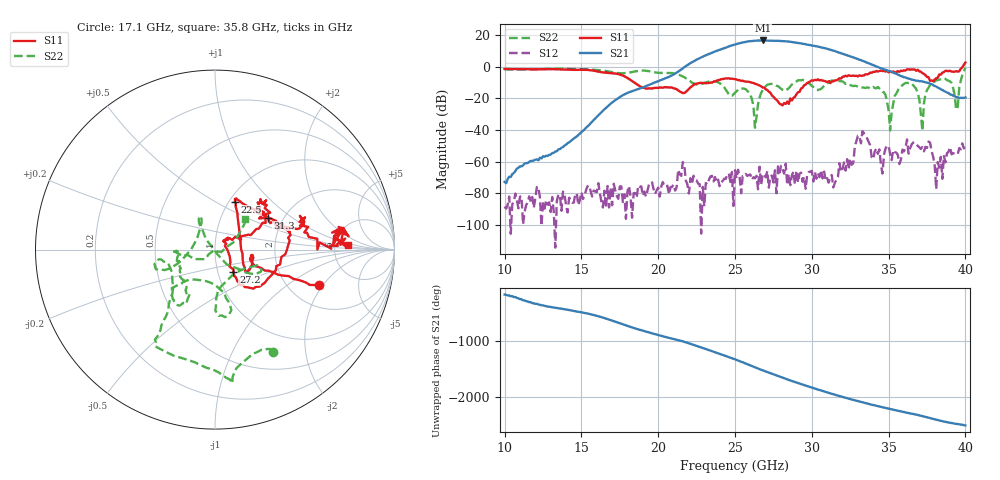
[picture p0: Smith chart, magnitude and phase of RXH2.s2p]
!Keysight Technologies,M9808A,MY58100618,A.14.70.03
!Date: Monday, February 27, 2023 13:24:29
!Correction: S11(Cdelta 2-Port  )
!S21(Cdelta 2-Port  )
!S12(Cdelta 2-Port  )
!S22(Cdelta 2-Port  )
!S2P File: Measurements: S11, S21, S12, S22:
# Hz S  RI  R 50
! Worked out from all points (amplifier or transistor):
!   301 points, 10 GHz to 40 GHz, reference 50 ohm
!   highest |S21| = 16.5 dB at 26.8 GHz (marker M1)
!   |S21| within 3 dB of that: 24.85 GHz to 29.92 GHz (5.075 GHz wide, 18.5 % of centre)
!   unconditionally stable (mu >= 1): start of sweep to 39.83 GHz
!   at 15 GHz: K = 61616.39, MAG = -31.9 dB, |S12| = -79.4 dB
!   at 25 GHz: K = 153.75, MAG = 14.8 dB, |S12| = -65.5 dB
!   at 40 GHz: K = -150.11, MSG = 15.3 dB, |S12| = -50.1 dB
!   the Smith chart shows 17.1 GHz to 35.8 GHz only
!   S11 on the Smith chart (normalised r, x): 17.1 GHz: 2.88, -1.83; 22.5 GHz: 1.06, +0.62; 27.2 GHz: 1.19, -0.30; 31.3 GHz: 1.66, +0.67; 35.8 GHz: 6.70, +0.69
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1e10  0.0322 0.8434  -0.000221 -6.08e-05  -3.66e-05 8.55e-06  0.7271 0.3718
1.5e10  0.7652 0.2163  -0.00457 -0.00715  -2.56e-05 -0.000104  0.6439 -0.5301
1.71e10  0.5788 -0.1988  0.0118 0.0791  -6.59e-05 -0.000187  0.3259 -0.5679
2e10  0.2093 -0.0348  -0.3381 -0.073  0.000108 0.000105  -0.1138 -0.6274
2.25e10  0.1096 0.2668  1.658 -0.0651  6.37e-05 -0.000245  -0.241 -0.1242
2.38e10  0.3124 0.1716  -1.75 -2.593  6.87e-05 -0.00021  -0.3124 -0.111
2.45e10  0.412 0.1003  -4.092 0.7685  -1.61e-05 0.000398  -0.1549 -0.0237
2.5e10  0.4032 0.0063  -2.385 4.394  -0.000377 0.000376  -0.0821 0.1245
2.55e10  0.3392 -0.1147  2.458 5.235  -0.000336 9.58e-05  -0.0826 0.186
2.6e10  0.2479 -0.2064  6.278 1.061  -0.000141 0.00036  -0.0698 0.1096
2.68e10  0.1336 -0.1733  1.353 -6.574  -3.2e-05 -0.000382  0.1416 -0.1116
2.72e10  0.1024 -0.125  -3.335 -5.764  0.000136 -6.13e-05  0.2453 -0.127
2.78e10  0.0761 -0.0213  -6.533 0.1143  -0.000466 0.000526  0.2234 -0.0898
2.86e10  0.0725 0.0667  -1.122 5.988  -0.000132 -0.000122  0.0158 -0.2354
2.93e10  0.1855 0.0833  4.386 3.151  0.000259 0.000363  0.0405 -0.3681
3e10  0.3075 0.2055  4.172 -2.064  0.000292 0.000416  0.0513 -0.2404
3.06e10  0.2528 0.2815  0.7761 -3.993  0.000523 -8.55e-05  -0.1074 -0.1669
3.13e10  0.2929 0.1782  -2.455 -2.219  0.00033 0.000181  -0.2354 -0.275
3.27e10  0.4984 0.1554  -0.7807 1.804  -0.000864 -0.000209  -0.1719 -0.1712
3.5e10  0.6528 0.0949  0.535 -0.4966  -0.00301 0.000927  -0.0344 -0.0252
3.58e10  0.7423 0.023  -0.0273 -0.5004  0.000492 0.00102  0.1669 0.1703
4e10  1.104 -0.7808  0.102 0.0308  -0.000998 0.00295  0.4635 -0.8149
